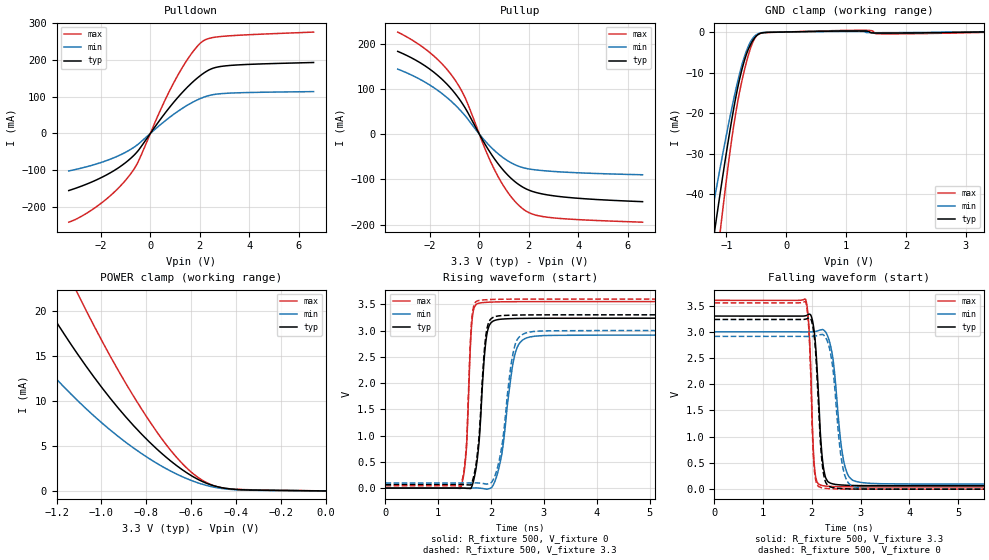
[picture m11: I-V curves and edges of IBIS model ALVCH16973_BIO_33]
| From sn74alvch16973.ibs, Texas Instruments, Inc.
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[Model]   ALVCH16973_BIO_33
Model_type  I/O
Vinl=0.8
Vinh=2.0
Enable   Active-Low
Vref =   0
Rref =   500
Cref =   50p
Vmeas =   1.5
| variable   typ   min   max
C_comp   3.09pF   2.74pF   3.41pF
| C_pullup   4.20pF   3.33pF   4.93pF
| C_pulldown   4.14pF   2.96pF   5.81pF
| C_tri-state   3.09pF   2.74pF   3.41pF
[Temperature Range]   40   100   -40
| Ambient temperature   25   85   -40
[Voltage range]   3.3   3   3.6
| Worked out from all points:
|   slope of the pulldown table from 0 to 0.495 V, typ, clamps not added: 10.7 ohm
|   slope of the pullup table from 0 to 0.495 V, typ, clamps not added: 10.9 ohm
|   GND clamp passes 1 mA (typ) near -0.50 V on its own axis
|   POWER clamp passes 1 mA (typ) near -0.55 V on its own axis
|   rising waveform, R_fixture 500, V_fixture 0: 20-80 % time 131ps typ, 217ps min, 85.5ps max; typ from 0 V to 3.23 V
|   falling waveform, R_fixture 500, V_fixture 3.3: 20-80 % time 120ps typ, 185ps min, 79.2ps max; typ from 3.3 V to 0.066 V
|   rising waveform, R_fixture 500, V_fixture 3.3: 20-80 % time 129ps typ, 206ps min, 84.9ps max; typ from 0.066 V to 3.3 V
|   falling waveform, R_fixture 500, V_fixture 0: 20-80 % time 117ps typ, 177ps min, 78.1ps max; typ from 3.23 V to 0 V
[GND Clamp]
| ALVCH16973_BIO_33
|   Voltage   I(typ)   I(min)   I(max)
-3.3V     -292.5mA   -240.9mA   -356.9mA
-1.285V   -58.1mA    -48.21mA   -72.65mA
-1.195V   -48.82mA   -40.75mA   -60.84mA
-1.165V   -45.78mA   -38.31mA   -56.96mA
-1.09V    -38.32mA   -32.32mA   -47.42mA
-915mV    -22.02mA   -19.13mA   -26.81mA
-790mV    -12.29mA   -10.87mA   -15.52mA
-620mV    -3.805mA   -3.097mA   -5.052mA
-480mV    -724.5uA   -513.5uA   -734.2uA
1.225V    241.9uA    133.4uA    415.4uA
1.57V     -286uA     -180.7uA   -464.8uA
3.3V      1.144nA    60.8uA     -106.7uA
[POWER Clamp]
| ALVCH16973_BIO_33
|   Voltage   I(typ)   I(min)   I(max)
-3.3V     143.6mA    105.5mA    167.4mA
-1.53V    33.24mA    22.37mA    45.78mA
-1.5V     31.81mA    21.37mA    43.97mA
-1.275V   21.8mA     14.48mA    30.94mA
-1.11V    15.37mA    10.14mA    22.17mA
-1.07V    13.94mA    9.187mA    20.17mA
-960mV    10.29mA    6.764mA    14.96mA
-785mV    5.416mA    3.563mA    7.735mA
-680mV    3.107mA    2.063mA    4.169mA
-590mV    1.562mA    1.075mA    1.89mA
-445mV    281.1uA    216.8uA    283.5uA
-48.03fV  1.144nA    2.341nA    157.4pA
[Pulldown]
| ALVCH16973_BIO_33
|   Voltage   I(typ)   I(min)   I(max)
-3.3V     -155.3mA   -102mA     -241.3mA
-1.92V    -117.9mA   -77.39mA   -186.1mA
-1.295V   -93.6mA    -60.93mA   -148.7mA
-780mV    -66.83mA   -42.71mA   -108.4mA
-475mV    -45.21mA   -28.32mA   -74.34mA
405mV     38.2mA     23.55mA    63.12mA
995mV     88.61mA    54.39mA    143.9mA
1.585V    131.4mA    80.05mA    209.4mA
2.08V     160mA      96.3mA     248.5mA
2.505V    176.4mA    104.9mA    260.1mA
3.03V     183.4mA    108.8mA    264.3mA
6.6V      192.6mA    113.5mA    275.2mA
[Pullup]
| ALVCH16973_BIO_33
|   Voltage   I(typ)   I(min)   I(max)
-3.3V     183mA      143.8mA    225.7mA
-2V       143.6mA    108.5mA    180.3mA
-1.48V    119.8mA    88.48mA    153.7mA
-1.04V    93.93mA    67.7mA     124.3mA
-550mV    55.76mA    39.02mA    77.44mA
245mV     -23.6mA    -15.83mA   -34.29mA
705mV     -61.65mA   -40.84mA   -88.44mA
1.23V     -94.91mA   -61.64mA   -134.7mA
1.755V    -117.1mA   -73.97mA   -165mA
2.185V    -127.4mA   -78.46mA   -177.5mA
2.86V     -135.3mA   -82.02mA   -184.5mA
6.6V      -149.4mA   -89.88mA   -194.8mA
[Ramp]
| ALVCH16973_BIO_33
| variable   typ   min   max
dV/dt_r   1.95/1.36E-10   1.76/2.24E-10   2.14/8.84E-11
dV/dt_f   1.96/1.26E-10   1.77/1.90E-10   2.15/8.23E-11
R_load = 500
[Rising Waveform]
| ALVCH16973_BIO_33
R_fixture =   500
C_fixture =   0
L_fixture =   0
V_fixture =   0
V_fixture_min = 0
V_fixture_max = 0
|   Time   V(typ)   V(min)   V(max)
0s        8.745nV    32.05nV    337.5pV
1.42ns    863.4uV    83.85uV    -8.659mV
1.535ns   -4.924mV   440.1uV    783.7mV
1.645ns   58.97mV    1.454mV    3.249V
1.82ns    1.669V     -5.512mV   3.531V
1.99ns    3.139V     -1.295mV   3.542V
2.205ns   3.219V     660mV      3.548V
2.465ns   3.23V      2.598V     3.55V
2.835ns   3.234V     2.894V     3.551V
29.99ns   3.235V     2.913V     3.552V
[Falling Waveform]
| ALVCH16973_BIO_33
R_fixture =   500
C_fixture =   0
L_fixture =   0
V_fixture =   3.3
V_fixture_min = 3
V_fixture_max = 3.6
|   Time   V(typ)   V(min)   V(max)
0s        3.3V       3V         3.6V
1.87ns    3.306V     2.998V     3.621V
1.945ns   3.337V     2.997V     3.006V
2.055ns   2.959V     3.003V     410.5mV
2.185ns   928.1mV    3.037V     76.27mV
2.255ns   326.8mV    3.024V     62.11mV
2.43ns    101.1mV    2.512V     50.1mV
2.675ns   76.15mV    448.9mV    45.78mV
3.035ns   68.02mV    124.2mV    44.17mV
29.99ns   66.45mV    96.86mV    43.74mV
[Rising Waveform]
| ALVCH16973_BIO_33
R_fixture =   500
C_fixture =   0
L_fixture =   0
V_fixture =   3.3
V_fixture_min = 3
V_fixture_max = 3.6
|   Time   V(typ)   V(min)   V(max)
0s        66.45mV    96.86mV    43.74mV
1.42ns    67.23mV    96.95mV    35.42mV
1.53ns    61.73mV    97.24mV    779.5mV
1.64ns    113mV      98.07mV    3.281V
1.8ns     1.413V     93.21mV    3.579V
1.96ns    3.168V     85.56mV    3.59V
2.18ns    3.283V     659.9mV    3.596V
2.45ns    3.295V     2.714V     3.599V
2.8ns     3.299V     2.982V     3.6V
29.99ns   3.3V       3V         3.6V
[Falling Waveform]
| ALVCH16973_BIO_33
R_fixture =   500
C_fixture =   0
L_fixture =   0
V_fixture =   0
V_fixture_min = 0
V_fixture_max = 0
|   Time   V(typ)   V(min)   V(max)
0s        3.235V     2.913V     3.552V
1.87ns    3.241V     2.911V     3.571V
1.945ns   3.271V     2.911V     2.927V
2.05ns    2.905V     2.917V     382.8mV
2.18ns    842.8mV    2.946V     33.24mV
2.25ns    249.3mV    2.93V      17.73mV
2.42ns    32.68mV    2.383V     6.272mV
2.655ns   9.371mV    336.2mV    2.103mV
3.01ns    1.465mV    21.99mV    451.2uV
29.99ns   19.26nV    104.7nV    371.5pV
